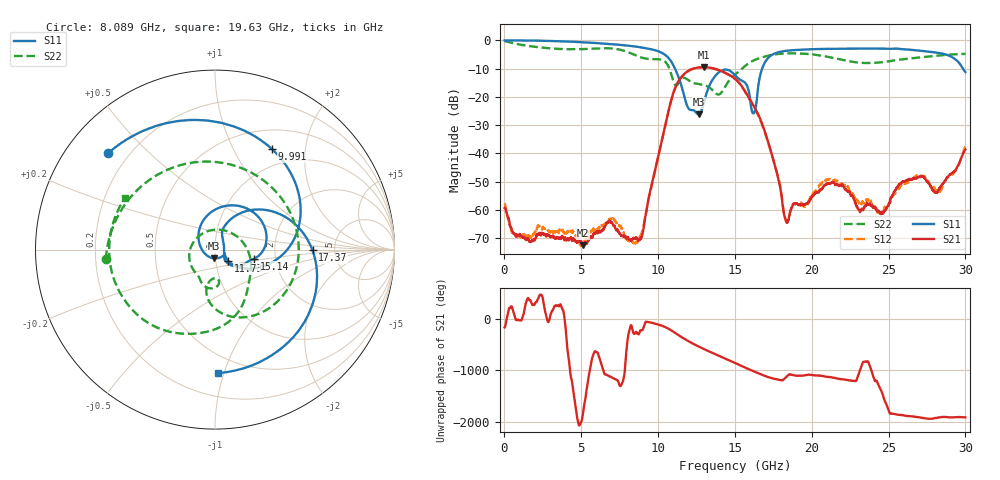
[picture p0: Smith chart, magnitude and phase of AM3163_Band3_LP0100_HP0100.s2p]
!Agilent Technologies,E8364B,MY43040894,A.07.50.67
!Agilent E8364B: A.07.50.67
!Date: Thursday, August 20, 2020 11:05:47
!Correction: S11(Full 2 Port(1,2))
!S21(Full 2 Port(1,2))
!S12(Full 2 Port(1,2))
!S22(Full 2 Port(1,2))
!S2P File: Measurements: S11, S21, S12, S22:
# Hz S  dB  R 50
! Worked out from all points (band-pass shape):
!   3201 points, 10 MHz to 30 GHz, reference 50 ohm
!   highest |S21| = -9.48 dB at 12.96 GHz (marker M1); lowest = -72.5 dB at 5.09 GHz (marker M2)
!   |S21| within 3 dB of the highest: 11.59 GHz to 14.71 GHz (3.119 GHz wide, 23.7 % of centre)
!   lowest |S11| = -26.2 dB at 12.63 GHz (marker M3), VSWR 1.10, Z = 49.3 - j4.83 ohm
!   |S11| at or under -10 dB: 11.1 GHz to 16.77 GHz (5.672 GHz wide, 40.7 % of centre); 29.84 GHz to end of sweep
!   |S22| runs from -19.2 to -0.3 dB; largest |S21 - S12| = 0.0037
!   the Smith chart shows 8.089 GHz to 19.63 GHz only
!   S11 on the Smith chart (normalised r, x): 8.089 GHz: 0.13, +0.38; 9.991 GHz: 0.75, +1.44; 11.73 GHz: 1.15, -0.14; 15.14 GHz: 1.54, -0.17; 17.37 GHz: 3.38, -0.04; 19.63 GHz: 0.36, -0.95
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1e7  -0.04 -2.0  -59.27 -172.3  -57.62 64.5  -0.28 -6.5
1.012791e9  -0.05 -27.7  -68.67 -36.8  -69.27 -136.8  -1.51 -85.3
2.315481e9  -0.13 -63.2  -68.51 102.0  -66.19 68.8  -2.50 -168.7
5.014581e9  -0.66 -134.8  -71.15 173.3  -72.50 -160.4  -3.12 47.9
5.089556e9  -0.68 -136.8  -72.52 -81.2  -72.15 90.0  -3.11 43.7
6.954559e9  -1.34 172.5  -64.40 -54.0  -62.98 -71.7  -2.85 -77.4
8.088556e9  -1.91 138.0  -70.04 84.3  -70.84 -175.2  -4.29 -175.0
9.991047e9  -3.83 60.4  -41.51 -113.0  -41.65 -113.7  -6.65 -13.6
1.000979e10  -3.86 59.4  -41.01 -114.8  -41.23 -115.3  -6.66 -15.6
1.173422e10  -20.40 -40.2  -11.72 -36.8  -11.81 -36.6  -13.31 -101.4
1.263392e10  -26.18 -95.4  -9.60 179.3  -9.66 179.7  -15.44 -129.4
1.296193e10  -22.33 175.4  -9.48 132.5  -9.54 132.8  -15.82 -142.8
1.5005e10  -12.32 -9.0  -13.57 -138.5  -13.66 -138.4  -12.14 -37.8
1.513621e10  -13.04 -13.3  -14.21 -156.8  -14.31 -156.7  -11.58 -44.2
1.622334e10  -25.77 9.2  -23.19 60.2  -23.44 60.5  -7.09 -89.4
1.736671e10  -5.30 -0.4  -39.68 -71.2  -39.82 -68.4  -5.17 -131.6
1.833202e10  -3.70 -47.6  -64.07 -53.4  -64.03 20.5  -4.62 -165.0
1.962533e10  -3.24 -88.8  -57.98 -15.0  -58.71 -16.1  -4.75 150.4
2.000958e10  -3.14 -99.1  -55.15 -11.2  -54.64 -7.4  -4.95 136.2
2.267119e10  -2.92 -161.2  -55.05 -125.8  -54.47 -133.7  -7.60 17.6
2.500479e10  -2.98 144.7  -57.87 22.2  -57.93 72.5  -7.44 -94.8
3e10  -11.22 -20.2  -38.61 -113.1  -37.61 -118.9  -4.78 103.0
